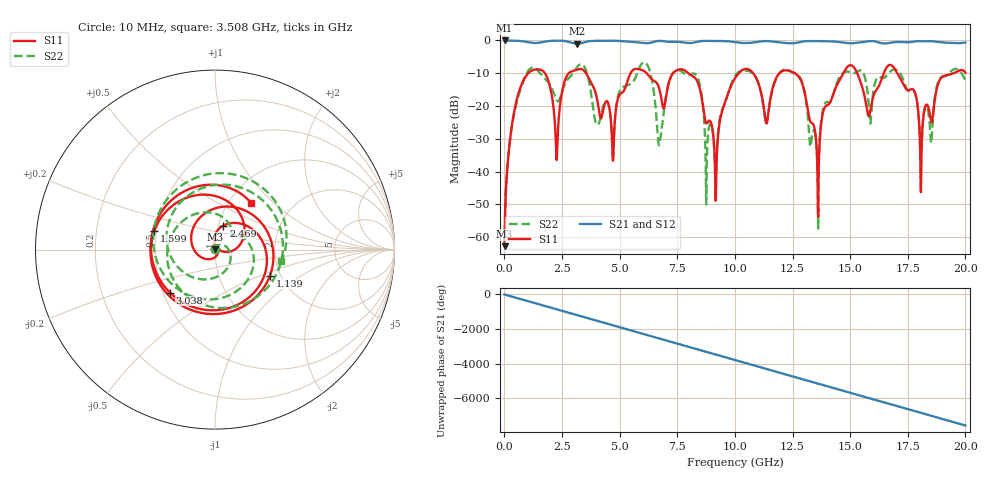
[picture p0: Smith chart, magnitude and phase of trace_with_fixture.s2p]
! Created with skrf 1.10.0 (http://scikit-rf.org).
# GHz S RI R 50.0
!freq ReS11 ImS11 ReS21 ImS21 ReS12 ImS12 ReS22 ImS22
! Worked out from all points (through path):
!   2001 points, 10 MHz to 20 GHz, reference 50 ohm
!   highest |S21| = 0.00 dB at 10 MHz (marker M1); lowest = -1.0 dB at 3.148 GHz (marker M2)
!   group delay of S21, straight-line fit = 1.05 ns
!   lowest |S11| = -62.7 dB at 10 MHz (marker M3), VSWR 1.00, Z = 50 + j0.0723 ohm
!   |S11| at or under -10 dB: 7.98 GHz to 10.17 GHz (2.187 GHz wide, 24.1 % of centre); 12.59 GHz to 14.71 GHz (2.114 GHz wide, 15.5 % of centre); 17.05 GHz to 19.48 GHz (2.438 GHz wide, 13.3 % of centre)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
!   |S22| runs from -62.7 to -6.6 dB; largest |S21 - S12| = 7e-16
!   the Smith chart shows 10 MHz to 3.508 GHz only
!   S11 on the Smith chart (normalised r, x): 10 MHz: 1.00, +0.00; 1.139 GHz: 1.76, -0.58; 1.599 GHz: 0.48, +0.12; 2.469 GHz: 1.06, +0.29; 3.038 GHz: 0.54, -0.30; 3.508 GHz: 1.26, +0.74
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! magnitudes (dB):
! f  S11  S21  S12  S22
! 10 MHz  -62.7  0.0  0.0  -62.7
! 399.8 MHz  -22.7  0.0  0.0  -23.2
! 1.139 GHz  -9.4  -0.6  -0.6  -8.5
! 1.599 GHz  -9.0  -0.6  -0.6  -10.4
! 2.259 GHz  -35.8  -0.1  -0.1  -18.1
! 2.469 GHz  -17.0  -0.1  -0.1  -16.5
! 3.038 GHz  -9.2  -0.9  -0.9  -9.3
! 3.148 GHz  -8.9  -1.0  -1.0  -8.2
! 3.348 GHz  -8.7  -0.8  -0.8  -7.2
! 3.508 GHz  -9.7  -0.5  -0.5  -8.5
! 4.708 GHz  -36.7  -0.1  -0.1  -36.9
! 6.137 GHz  -9.8  -0.8  -0.8  -6.9
! 6.677 GHz  -13.8  -0.1  -0.1  -30.9
! 8.236 GHz  -11.2  -0.6  -0.6  -10.1
! 9.165 GHz  -48.9  -0.1  -0.1  -47.1
! 10.01 GHz  -11.5  -0.5  -0.5  -10.8
! 11.36 GHz  -25.3  -0.2  -0.2  -25.6
! 12.71 GHz  -10.6  -0.7  -0.7  -10.4
! 13.34 GHz  -25.2  -0.2  -0.2  -29.3
! 16.67 GHz  -7.6  -0.8  -0.8  -10.0
! 18.08 GHz  -39.9  -0.2  -0.2  -37.5
! 20 GHz  -9.8  -0.6  -0.6  -12.2
